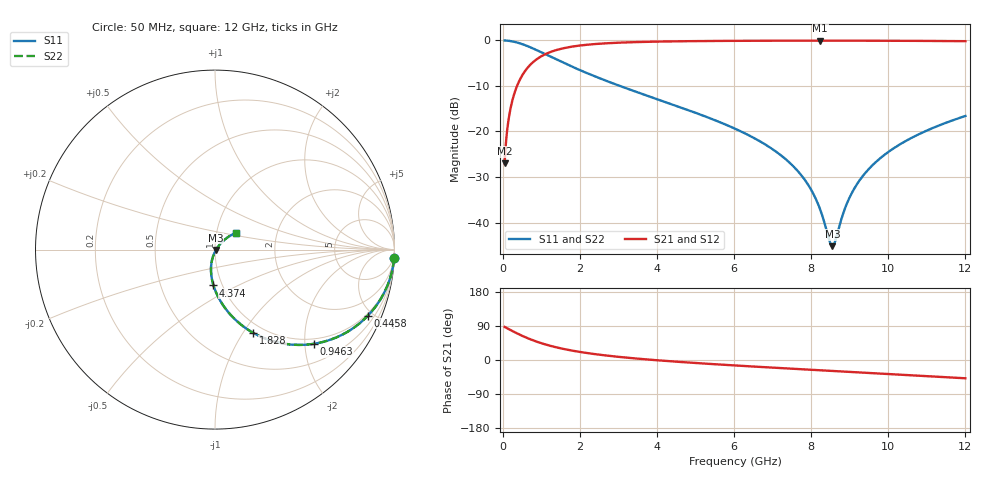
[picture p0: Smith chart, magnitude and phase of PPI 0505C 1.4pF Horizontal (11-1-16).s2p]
# MHz S MA R 50
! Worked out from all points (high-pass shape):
!   1601 points, 50 MHz to 12 GHz, reference 50 ohm
!   highest |S21| = -0.05 dB at 8.236 GHz (marker M1); lowest = -27.0 dB at 50 MHz (marker M2)
!   |S21| within 3 dB of the highest: 1.098 GHz to end of sweep
!   lowest |S11| = -45.2 dB at 8.549 GHz (marker M3), VSWR 1.01, Z = 50.5 - j0.277 ohm
!   |S11| at or under -10 dB: 3.04 GHz to end of sweep
!   |S22| runs from -45.2 to 0.0 dB; largest |S21 - S12| = 0
!   S11 on the Smith chart (normalised r, x): 50 MHz: 1, -42; 445.8 MHz: 0.88, -4.69; 946.2 MHz: 0.88, -2.19; 1.828 GHz: 0.89, -1.11; 4.374 GHz: 0.91, -0.38; 12 GHz: 1.24, +0.23
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50  0.999 -2.7  0.04464 87.3  0.04464 87.3  0.999 -2.7
147.0938  0.9914 -8.0  0.1303 82.0  0.1303 82.0  0.9914 -8.0
206.8438  0.9833 -11.2  0.1818 78.8  0.1818 78.8  0.9833 -11.2
445.8438  0.9285 -23.3  0.3706 66.7  0.3706 66.7  0.9285 -23.3
946.25  0.7602 -43.7  0.6482 46.2  0.6482 46.2  0.7602 -43.7
1827.562  0.5089 -65.5  0.8584 24.3  0.8584 24.3  0.5089 -65.5
2044.156  0.4641 -69.1  0.8831 20.6  0.8831 20.6  0.4641 -69.1
2880.656  0.335 -79.8  0.939 9.6  0.939 9.6  0.335 -79.8
4038.312  0.2239 -90.0  0.9708 -0.9  0.9708 -0.9  0.2239 -90.0
4374.406  0.1997 -92.4  0.9759 -3.5  0.9759 -3.5  0.1997 -92.4
6025  0.1073 -102.1  0.9894 -14.4  0.9894 -14.4  0.1073 -102.1
7272.281  0.05242 -106.3  0.9932 -21.7  0.9932 -21.7  0.05242 -106.3
8019.156  0.02215 -102.2  0.994 -25.9  0.994 -25.9  0.02215 -102.2
8235.75  0.01384 -94.3  0.994 -27.1  0.994 -27.1  0.01384 -94.3
8474.75  0.006293 -58.1  0.994 -28.4  0.994 -28.4  0.006293 -58.1
8549.438  0.005504 -29.9  0.994 -28.9  0.994 -28.9  0.005504 -29.9
8624.125  0.006257 -1.5  0.9939 -29.3  0.9939 -29.3  0.006257 -1.5
8907.938  0.01545 37.6  0.9937 -30.8  0.9937 -30.8  0.01545 37.6
9146.938  0.02474 44.3  0.9934 -32.2  0.9934 -32.2  0.02474 44.3
9520.375  0.03975 47.1  0.9927 -34.2  0.9927 -34.2  0.03975 47.1
10013.31  0.06006 47.1  0.9914 -37.0  0.9914 -37.0  0.06006 47.1
12000  0.1481 38.9  0.9809 -48.3  0.9809 -48.3  0.1481 38.9
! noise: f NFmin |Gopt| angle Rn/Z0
50  0.0009862  0.9602  1.669  0.005588
1372  0.005843  0.768  6.368  0.005111
2701  0.009229  0.7178  10.54  0.006415
4031  0.01222  0.6884  14.79  0.007504
5360  0.01504  0.6691  19.01  0.008508
6682  0.01778  0.6564  23.15  0.009488
8012  0.02053  0.6485  27.24  0.0105
9341  0.02333  0.6445  31.23  0.01157
1.067e+04  0.02624  0.6438  35.12  0.01273
1.2e+04  0.0293  0.6461  38.91  0.01403
